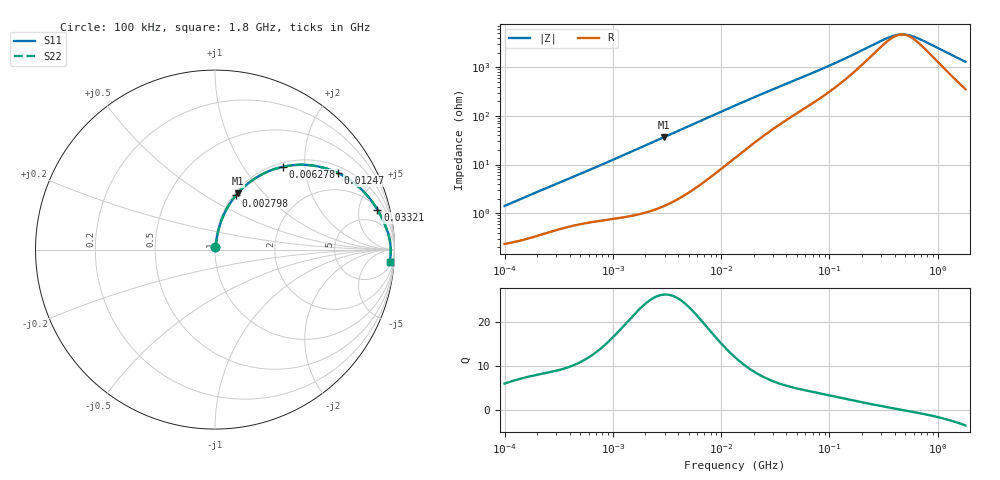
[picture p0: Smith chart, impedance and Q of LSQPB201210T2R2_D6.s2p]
! LSQPB201210T2R2_D6  S-PARAMETER MODEL  ( General Type )
! Model Generated by TAIYO YUDEN Corporation (http://www.ty-top.com)
! Version 1.0
! TAIYO YUDEN Control No. 120417NG38SB-FKC
! Copyright(c) 2012 TAIYO YUDEN CO.,LTD. All Rights Reserved.
! Product Description (link to TY-COMPAS)
! https://ds.yuden.co.jp/TYCOMPAS/or/detail?pn=LSQPB201210T2R2MD6&u=M
! Products Name : Inductors
! Characteristics :
!  Inductance : 2.2 uH , SRF(min) : 250 MHz , DC Resistance(max) : 0.2392 Ohm
!  Rated Current : Saturation :680 mA , Temp Rise : 950 mA (40 degC)
!  Case Size : 2.0 x 1.25 / 0.079 x 0.049 [mm/inch] , Thickness : 1.0 / 0.04 [mm/inch]
!  (Conditions: Temperature = 25 degC , DC Bias Current/Voltage = 0A / 0V)
! External Node Assignments :
!  1  o---GGG---o  2
! GND o---------o GND
! Frequency Range : 0.1MHz  -  1800MHz  [ 402 STEP ]
# MHz S RI R 50
! Freq[MHz].  S11 Real  S11 Imag  S21 Real  S21 Imag  S12 Real  S12 Imag  S22 Real  S22 Imag
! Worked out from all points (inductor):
!   401 points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, 100 kHz to 1.8 GHz, reference 50 ohm
!   read as one part in series: L = 2.2 uH near 105 kHz
!   highest Q = 26.1 at 2.938 MHz (marker M1), where L = 1.97 uH
!   self-resonance near 466.6 MHz
!   S11 on the Smith chart (normalised r, x): 100 kHz: 1.00, +0.03; 2.798 MHz: 1.03, +0.69; 6.278 MHz: 1.07, +1.54; 12.47 MHz: 1.24, +3.03; 33.21 MHz: 2.25, +7.61; 1.8 GHz: 8, -25
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0.1  0.00253 0.0139  0.9975 -0.0139  0.9975 -0.0139  0.00253 0.0139
0.516129  0.0103 0.0651  0.9897 -0.0651  0.9897 -0.0651  0.0103 0.0651
1.216451  0.03 0.1458  0.97 -0.1458  0.97 -0.1458  0.03 0.1458
1.890522  0.0604 0.2179  0.9396 -0.2179  0.9396 -0.2179  0.0604 0.2179
2.66389  0.107 0.2904  0.893 -0.2904  0.893 -0.2904  0.107 0.2904
2.797645  0.116 0.3016  0.884 -0.3016  0.884 -0.3016  0.116 0.3016
2.938117  0.1258 0.313  0.8742 -0.313  0.8742 -0.313  0.1258 0.313
4.242694  0.2244 0.3975  0.7756 -0.3975  0.7756 -0.3975  0.2244 0.3975
6.278453  0.3798 0.4618  0.6202 -0.4618  0.6202 -0.4618  0.3798 0.4618
8.632747  0.5274 0.4703  0.4726 -0.4703  0.4726 -0.4703  0.5274 0.4703
12.46584  0.6848 0.4267  0.3152 -0.4267  0.3152 -0.4267  0.6848 0.4267
13.41641  0.7117 0.4129  0.2883 -0.4129  0.2883 -0.4129  0.7117 0.4129
20.3463  0.8293 0.3223  0.1707 -0.3223  0.1707 -0.3223  0.8293 0.3223
33.20848  0.9051 0.2223  0.0949 -0.2223  0.0949 -0.2223  0.9051 0.2223
69.24595  0.955 0.1185  0.045 -0.1185  0.045 -0.1185  0.955 0.1185
134.1607  0.9722 0.0609  0.0278 -0.0609  0.0278 -0.0609  0.9722 0.0609
357.3983  0.9789 0.0106  0.0211 -0.0106  0.0211 -0.0106  0.9789 0.0106
456.5984  0.9792 0.000853  0.0208 -0.000853  0.0208 -0.000853  0.9792 0.000853
516.0898  0.9793 -0.00397  0.0207 0.00397  0.0207 0.00397  0.9793 -0.00397
583.3325  0.9793 -0.00885  0.0207 0.00885  0.0207 0.00885  0.9793 -0.00885
727.2099  0.9791 -0.018  0.0209 0.018  0.0209 0.018  0.9791 -0.018
1800  0.9745 -0.0705  0.0255 0.0705  0.0255 0.0705  0.9745 -0.0705
